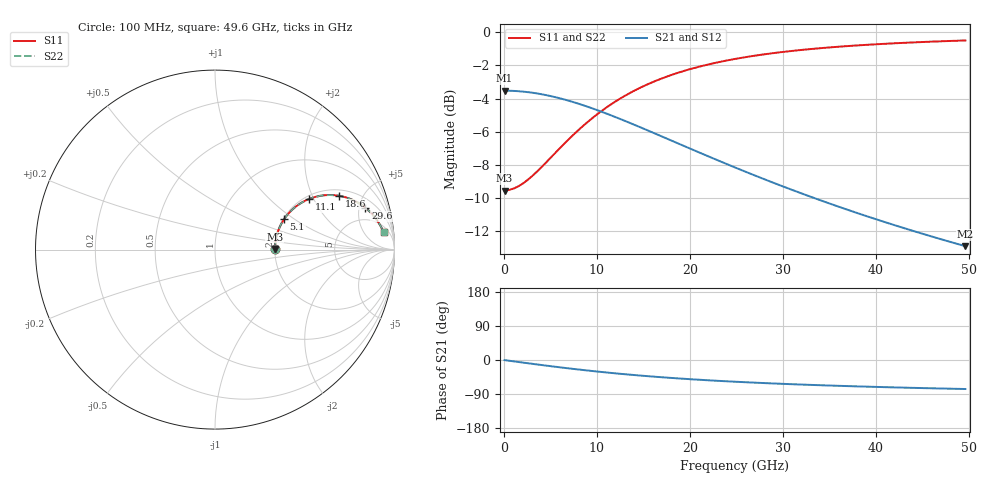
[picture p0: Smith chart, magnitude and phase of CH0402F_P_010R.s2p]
# GHz S RI R 10
! S-Parameters data
! Freq  reS11  imS11  reS21  imS21  reS12  imS12  reS22  imS22
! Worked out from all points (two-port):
!   100 points, 100 MHz to 49.6 GHz, reference 10 ohm
!   highest |S21| = -3.52 dB at 100 MHz (marker M1); lowest = -12.9 dB at 49.6 GHz (marker M2)
!   |S21| within 3 dB of the highest: start of sweep to 17.99 GHz
!   lowest |S11| = -9.5 dB at 100 MHz (marker M3), VSWR 2.00, Z = 20 + j0.162 ohm
!   |S11| at or under -10 dB: nowhere
!   |S22| runs from -9.5 to -0.5 dB; largest |S21 - S12| = 0
!   S11 on the Smith chart (normalised r, x): 100 MHz: 2.00, +0.02; 5.1 GHz: 2.02, +0.83; 11.1 GHz: 2.11, +1.84; 18.6 GHz: 2.33, +3.23; 29.6 GHz: 3.02, +5.78; 49.6 GHz: 8, +15
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0.1  0.3334 0.0036  0.6666 -0.00385  0.6666 -0.00385  0.3334 0.0036
1.1  0.3359 0.0394  0.6641 -0.0422  0.6641 -0.0422  0.3359 0.0394
2.1  0.3426 0.0744  0.6574 -0.0797  0.6574 -0.0797  0.3426 0.0744
3.6  0.3599 0.1241  0.6401 -0.1332  0.6401 -0.1332  0.3599 0.1241
5.1  0.3846 0.1688  0.6153 -0.1817  0.6153 -0.1817  0.3846 0.1688
7.1  0.4263 0.2186  0.5735 -0.2365  0.5735 -0.2365  0.4263 0.2186
8.6  0.4617 0.2479  0.538 -0.2696  0.538 -0.2696  0.4617 0.2479
9.6  0.4863 0.2637  0.5134 -0.2878  0.5134 -0.2878  0.4863 0.2637
11.1  0.5237 0.2818  0.4759 -0.3097  0.4759 -0.3097  0.5237 0.2818
12.1  0.5485 0.2906  0.4511 -0.321  0.4511 -0.321  0.5485 0.2906
13.6  0.5846 0.2993  0.4149 -0.3335  0.4149 -0.3335  0.5846 0.2993
15.1  0.6189 0.3035  0.3804 -0.3414  0.3804 -0.3414  0.6189 0.3035
16.6  0.6511 0.3039  0.348 -0.3456  0.348 -0.3456  0.6511 0.3039
18.6  0.6904 0.2998  0.3085 -0.3466  0.3085 -0.3466  0.6904 0.2998
21.6  0.7414 0.2867  0.2572 -0.341  0.2572 -0.341  0.7414 0.2867
25.1  0.7898 0.2652  0.2082 -0.3282  0.2082 -0.3282  0.7898 0.2652
27.1  0.8128 0.2513  0.1849 -0.3193  0.1849 -0.3193  0.8128 0.2513
29.6  0.8376 0.2331  0.1597 -0.3074  0.1597 -0.3074  0.8376 0.2331
33.1  0.866 0.2073  0.1306 -0.2904  0.1306 -0.2904  0.866 0.2073
37.1  0.8914 0.1783  0.1043 -0.2714  0.1043 -0.2714  0.8914 0.1783
41.6  0.9131 0.1471  0.0814 -0.2514  0.0814 -0.2514  0.9131 0.1471
49.6  0.9396 0.0962  0.0527 -0.2204  0.0527 -0.2204  0.9396 0.0962
